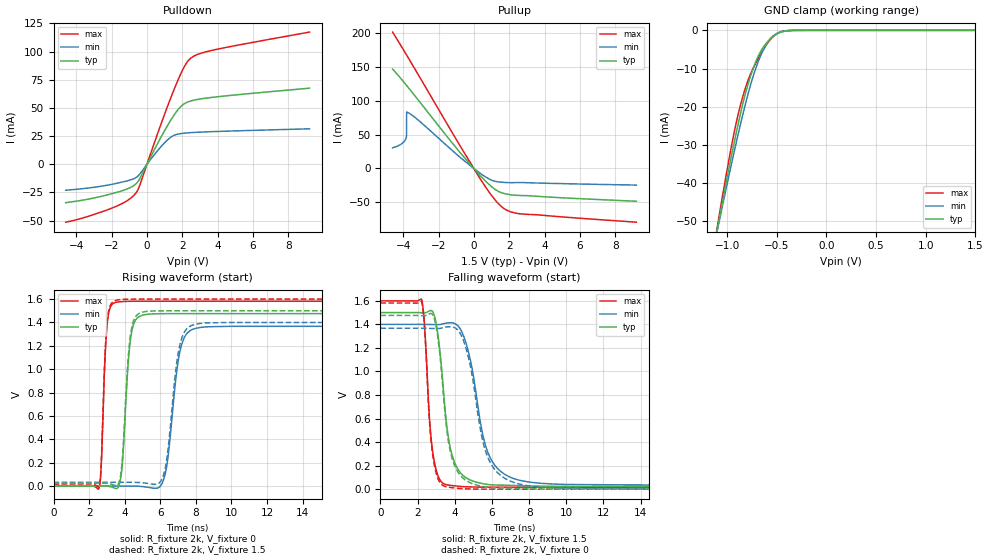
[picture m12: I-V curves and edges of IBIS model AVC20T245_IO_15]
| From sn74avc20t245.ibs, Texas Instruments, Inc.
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[Model]   AVC20T245_IO_15
Model_type  I/O
Vinl=0.49
Vinh=1.04
Enable   Active-Low
Vref =   0
Rref =   2000
Cref =   15p
Vmeas =   0.75
| variable   typ   min   max
C_comp   5.18pF   4.55pF   5.77pF
| C_pullup   5.10pF   3.65pF   7.53pF
| C_pulldown   4.79pF   4.27pF   5.46pF
| C_tri-state   5.18pF   4.55pF   5.77pF
[Temperature Range]   40   100   -40
| Ambient temperature   25   85   -40
[Voltage range]   1.5   1.4   1.6
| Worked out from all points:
|   slope of the pulldown table from 0 to 0.225 V, typ, clamps not added: 32.1 ohm
|   slope of the pullup table from 0 to 0.225 V, typ, clamps not added: 33.9 ohm
|   GND clamp passes 1 mA (typ) near -0.50 V on its own axis
|   rising waveform, R_fixture 2k, V_fixture 0: 20-80 % time 355ps typ, 580ps min, 237ps max; typ from 0 V to 1.48 V
|   falling waveform, R_fixture 2k, V_fixture 1.5: 20-80 % time 628ps typ, 1ns min, 383ps max; typ from 1.5 V to 0.023 V
|   rising waveform, R_fixture 2k, V_fixture 1.5: 20-80 % time 351ps typ, 568ps min, 235ps max; typ from 0.023 V to 1.5 V
|   falling waveform, R_fixture 2k, V_fixture 0: 20-80 % time 629ps typ, 998ps min, 376ps max; typ from 1.48 V to 0 V
[GND Clamp]
| AVC20T245_IO_15
|   Voltage   I(typ)   I(min)   I(max)
-4.6V     -597.8mA   -546.6mA   -662.5mA
-1.1V     -52.11mA   -52.52mA   -51.59mA
-1.075V   -48.66mA   -49.4mA    -47.7mA
-930mV    -29.5mA    -31.88mA   -26.82mA
-830mV    -17.94mA   -20.74mA   -16.24mA
-765mV    -12.02mA   -14.35mA   -11.48mA
-685mV    -6.644mA   -8.056mA   -7.261mA
-605mV    -3.35mA    -3.664mA   -3.806mA
-535mV    -1.602mA   -1.422mA   -1.608mA
-460mV    -500.6uA   -413.1uA   -383.6uA
-350mV    -38.76uA   -40.58uA   -15.38uA
1.5V      804.6pA    34.44nA    79.67pA
[Pulldown]
| AVC20T245_IO_15
|   Voltage   I(typ)   I(min)   I(max)
-4.6V     -34.07mA   -23.01mA   -51.35mA
-1.885V   -25.62mA   -17.44mA   -38.24mA
-1.09V    -21.68mA   -14.59mA   -31.97mA
-630mV    -17.39mA   -11.88mA   -25.55mA
-415mV    -12.94mA   -8.777mA   -18.95mA
595mV     18.22mA    11.97mA    26.91mA
1.265V    37.01mA    23.01mA    55.56mA
1.7V      47.29mA    26.56mA    72.61mA
2.03V     52.78mA    27.45mA    84.03mA
2.5V      56.24mA    28.09mA    94.31mA
3.84V     59.63mA    29.04mA    101.6mA
9.2V      67.51mA    31.46mA    117.2mA
[Pullup]
| AVC20T245_IO_15
|   Voltage   I(typ)   I(min)   I(max)
-4.6V     146.8mA    30.47mA    201.5mA
-4.1V     131.8mA    36.24mA    180.2mA
-3.85V    123.9mA    43.96mA    169.4mA
-3.81V    122.6mA    49.37mA    167.6mA
-3.805V   122.5mA    83.3mA     167.4mA
-3.785V   121.8mA    83.17mA    166.5mA
-3.155V   101.3mA    71.56mA    138.8mA
175mV     -5.197mA   -3.574mA   -7.497mA
980mV     -26.35mA   -16.94mA   -39.04mA
1.625V    -36.35mA   -20.39mA   -57.65mA
2.595V    -39.89mA   -20.78mA   -66.9mA
9.2V      -48.41mA   -24.54mA   -79.36mA
[Ramp]
| AVC20T245_IO_15
| variable   typ   min   max
dV/dt_r   0.90/3.68E-10   0.83/5.92E-10   0.96/2.50E-10
dV/dt_f   0.90/6.38E-10   0.83/1.01E-09   0.96/3.92E-10
R_load = 2k
[Rising Waveform]
| AVC20T245_IO_15
R_fixture =   2k
C_fixture =   0
L_fixture =   0
V_fixture =   0
V_fixture_min = 0
V_fixture_max = 0
|   Time   V(typ)   V(min)   V(max)
0s        19.4nV     97.73nV    508.8pV
2.565ns   916.4uV    -148.7uV   -15.7mV
3ns       -110.7uV   138.2uV    1.36V
3.5ns     -20.62mV   673.8uV    1.571V
4.365ns   1.296V     539.7uV    1.581V
5.015ns   1.463V     -3.912mV   1.582V
6.19ns    1.475V     56.84mV    1.582V
7.1ns     1.475V     1.149V     1.582V
7.985ns   1.475V     1.349V     1.582V
40ns      1.476V     1.367V     1.582V
[Falling Waveform]
| AVC20T245_IO_15
R_fixture =   2k
C_fixture =   0
L_fixture =   0
V_fixture =   1.5
V_fixture_min = 1.4
V_fixture_max = 1.6
|   Time   V(typ)   V(min)   V(max)
0s        1.5V       1.4V       1.6V
2.21ns    1.499V     1.4V       1.615V
2.805ns   1.51V      1.398V     328.3mV
3.13ns    1.269V     1.398V     103.1mV
3.55ns    567.8mV    1.411V     38.26mV
3.92ns    256.8mV    1.411V     29.63mV
4.57ns    101.1mV    1.259V     20.76mV
5.88ns    38.33mV    275.9mV    17.36mV
7.505ns   29.64mV    74.67mV    17.21mV
40ns      23.49mV    32.45mV    17.19mV
[Rising Waveform]
| AVC20T245_IO_15
R_fixture =   2k
C_fixture =   0
L_fixture =   0
V_fixture =   1.5
V_fixture_min = 1.4
V_fixture_max = 1.6
|   Time   V(typ)   V(min)   V(max)
0s        23.49mV    32.45mV    17.19mV
2.56ns    24.39mV    32.33mV    -123.5uV
3.005ns   23.22mV    32.62mV    1.393V
3.525ns   2.906mV    33.14mV    1.59V
4.335ns   1.302V     32.84mV    1.599V
4.995ns   1.488V     28.68mV    1.6V
6.175ns   1.5V       91.38mV    1.6V
7.065ns   1.5V       1.184V     1.6V
7.93ns    1.5V       1.383V     1.6V
40ns      1.5V       1.4V       1.6V
[Falling Waveform]
| AVC20T245_IO_15
R_fixture =   2k
C_fixture =   0
L_fixture =   0
V_fixture =   0
V_fixture_min = 0
V_fixture_max = 0
|   Time   V(typ)   V(min)   V(max)
0s        1.476V     1.367V     1.582V
2.21ns    1.474V     1.367V     1.596V
2.8ns     1.485V     1.365V     308mV
3.125ns   1.246V     1.365V     79.68mV
3.53ns    563mV      1.377V     20.86mV
3.905ns   239mV      1.377V     11.79mV
4.55ns    80.13mV    1.227V     3.269mV
5.84ns    14.69mV    248.8mV    160.6uV
7.5ns     5.655mV    42.02mV    16.41uV
40ns      21.17nV    529.2nV    28.82nV
